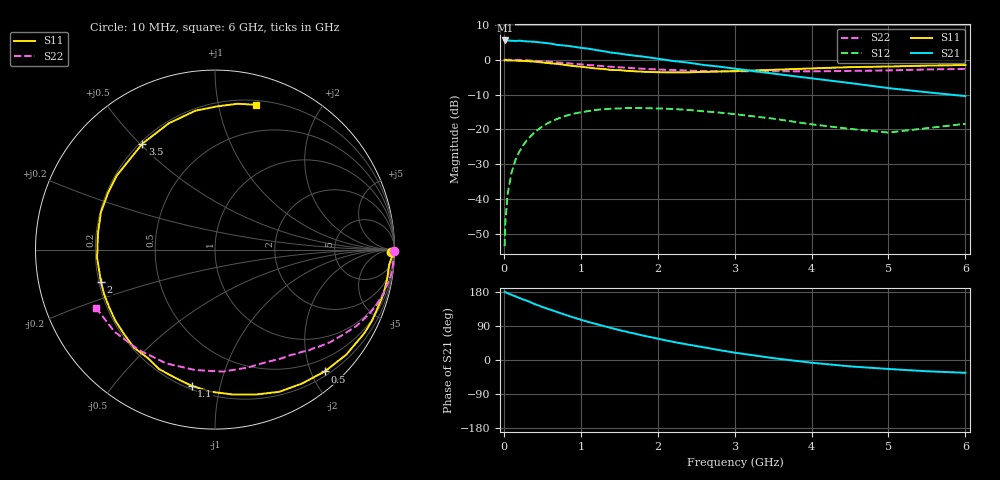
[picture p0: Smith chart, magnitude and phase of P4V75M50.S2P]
! SIEMENS Small Signal Semiconductors
! BFP182
! Si NPN RF Bipolar Junction Transistor in SOT143
! VCE = 0.75 V  IC = 0.5 mA
! Common Emitter S-Parameters:  March  1996
# GHz  S  MA  R  50
!  f  S11  S21  S12  S22
! GHz  MAG  ANG  MAG  ANG  MAG  ANG  MAG  ANG
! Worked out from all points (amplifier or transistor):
!   36 points, 10 MHz to 6 GHz, reference 50 ohm
!   highest |S21| = 5.5 dB at 20 MHz (marker M1)
!   |S21| within 3 dB of that: start of sweep to 1.272 GHz
!   unconditionally stable (mu >= 1): 2.792 GHz to end of sweep
!   at 250 MHz: K = 0.10, MSG = 15.0 dB, |S12| = -24.7 dB
!   at 1.4 GHz: K = 0.55, MSG = 8.1 dB, |S12| = -14.1 dB
!   at 6 GHz: K = 1.50, MAG = -0.2 dB, |S12| = -18.4 dB
!   S11 on the Smith chart (normalised r, x): 10 MHz: 62, -49; 500 MHz: 0.27, -2.22; 1.1 GHz: 0.22, -0.82; 2 GHz: 0.21, -0.13; 3.5 GHz: 0.21, +0.51; 6 GHz: 0.24, +1.29
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0.01  0.9804 -0.9  1.884 179.7  0.0021 87.9  0.9991 -0.4
0.02  0.9873 -2.2  1.889 179.1  0.0047 89.0  0.9993 -0.7
0.05  0.9742 -4.9  1.885 176.0  0.012 88.5  0.9983 -2.0
0.1  0.973 -9.7  1.872 171.9  0.0239 83.2  0.995 -3.9
0.15  0.9711 -14.8  1.855 168.0  0.036 80.1  0.9947 -5.9
0.2  0.9628 -19.7  1.876 163.7  0.0475 77.5  0.992 -7.8
0.3  0.9539 -29.1  1.831 156.4  0.07 70.4  0.979 -11.7
0.4  0.9369 -38.6  1.807 147.7  0.0908 64.5  0.9667 -15.4
0.5  0.9137 -48.0  1.759 140.0  0.1098 58.3  0.9508 -19.0
0.6  0.8895 -57.1  1.709 133.0  0.1275 52.3  0.9324 -22.3
0.8  0.8392 -74.2  1.592 119.2  0.1555 41.6  0.8954 -28.4
1.1  0.7704 -99.7  1.439 100.2  0.1832 27.6  0.8383 -36.2
1.5  0.7088 -129.7  1.228 79.0  0.1994 12.1  0.7768 -45.0
1.8  0.6721 -151.0  1.112 64.9  0.2021 3.0  0.7428 -50.5
2  0.6606 -164.1  1.034 56.4  0.1997 -2.4  0.7235 -54.2
2.2  0.6584 -176.0  0.959 47.8  0.1958 -7.8  0.7115 -58.2
2.8  0.6745 152.0  0.796 26.1  0.1742 -19.8  0.6832 -70.1
3.5  0.7156 124.4  0.632 5.0  0.1424 -28.1  0.6812 -86.2
4.5  0.7817 98.0  0.462 -16.8  0.1014 -22.9  0.6899 -113.2
5  0.7981 89.1  0.391 -23.7  0.0899 -10.2  0.7019 -127.0
5.5  0.8219 81.3  0.341 -29.7  0.1039 -0.1  0.7233 -140.8
6  0.8383 74.3  0.3 -33.8  0.1199 3.7  0.7376 -153.9
